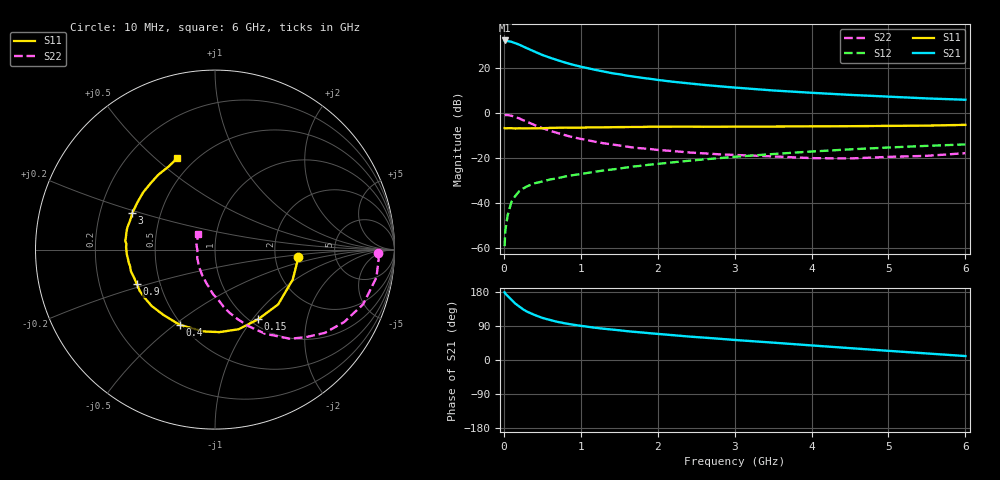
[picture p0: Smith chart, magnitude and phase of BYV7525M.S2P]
! SIEMENS Small Signal Semiconductors
! BFY420
! Si NPN RF SIEGET Grounded Emitter Transistor in MICRO-X
! VCE = 0.75 V  IC = 25 mA
! Common Emitter S-Parameters:  October  1996
# GHz  S  MA  R  50
!  f  S11  S21  S12  S22
! GHz  MAG  ANG  MAG  ANG  MAG  ANG  MAG  ANG
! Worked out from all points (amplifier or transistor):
!   36 points, 10 MHz to 6 GHz, reference 50 ohm
!   highest |S21| = 32.4 dB at 10 MHz (marker M1)
!   |S21| within 3 dB of that: start of sweep to 271 MHz
!   unconditionally stable (mu >= 1): start of sweep to 13.38 MHz; 1.469 GHz to end of sweep
!   at 250 MHz: K = 0.37, MSG = 31.6 dB, |S12| = -33.6 dB
!   at 1.4 GHz: K = 0.99, MSG = 21.5 dB, |S12| = -25.1 dB
!   at 6 GHz: K = 1.10, MAG = 8.0 dB, |S12| = -13.9 dB
!   S11 on the Smith chart (normalised r, x): 10 MHz: 2.71, -0.29; 150 MHz: 1.09, -1.07; 400 MHz: 0.49, -0.52; 900 MHz: 0.37, -0.18; 3 GHz: 0.34, +0.19; 6 GHz: 0.40, +0.59
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0.01  0.4659 -5.1  41.72 178.5  0.0011 103.7  0.91 -1.3
0.02  0.4626 -9.2  41.63 175.1  0.0025 81.3  0.9134 -3.4
0.05  0.4642 -21.1  40.42 168.8  0.0054 81.4  0.9125 -9.8
0.1  0.4658 -40.9  38.89 159.0  0.0108 75.6  0.8797 -20.3
0.15  0.4566 -58.1  36.19 148.8  0.0145 69.0  0.8249 -29.3
0.2  0.4629 -73.4  33.66 141.2  0.0183 66.1  0.7677 -37.2
0.25  0.4604 -86.9  30.69 133.7  0.021 61.1  0.7009 -44.2
0.3  0.4604 -98.2  28.02 127.8  0.0236 59.2  0.6481 -50.0
0.4  0.463 -115.2  23.55 118.8  0.0276 55.0  0.5459 -59.2
0.5  0.4636 -128.1  19.87 111.2  0.0303 54.2  0.4671 -66.2
0.6  0.4722 -138.1  17.23 105.6  0.0335 53.7  0.4082 -71.9
0.7  0.4754 -145.5  15.14 100.5  0.0359 53.6  0.3622 -76.9
0.9  0.4761 -156.3  12 93.1  0.0419 53.4  0.292 -84.7
1.1  0.4837 -165.4  9.993 87.4  0.0472 54.5  0.2493 -92.3
1.4  0.4885 -174.6  7.839 80.5  0.0558 54.6  0.2034 -101.4
1.6  0.4934 -179.1  6.882 76.1  0.0623 54.7  0.1808 -107.9
2.2  0.5029 169.1  5.022 65.5  0.0809 52.3  0.144 -123.7
3  0.5043 156.3  3.733 52.9  0.1073 47.6  0.1181 -142.4
3.5  0.506 148.5  3.215 45.8  0.1237 44.0  0.1095 -154.7
4.5  0.5147 134.4  2.566 31.3  0.1571 34.6  0.0985 -179.3
5.5  0.5307 118.9  2.139 17.3  0.188 24.4  0.1128 150.3
6  0.5515 112.4  1.997 10.4  0.2024 19.1  0.1293 138.1
